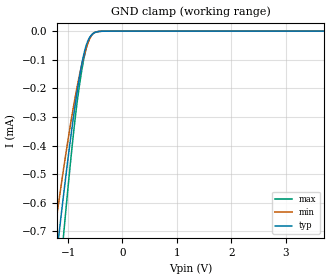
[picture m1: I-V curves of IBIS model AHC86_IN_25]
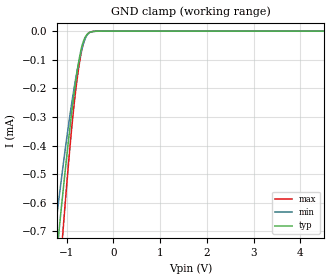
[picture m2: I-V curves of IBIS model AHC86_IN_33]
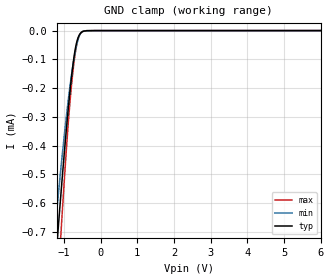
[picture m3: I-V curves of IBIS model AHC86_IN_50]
| TEXAS INSTRUMENTS INCORPORATED
| Standard Linear and Logic Group
| IBIS Model of SN74AHC86
| QUADRUPLE 2-INPUT EXCLUSIVE-OR GATES
| This file contains package information for the following:
|  SOIC 14-pin (D) package as [Component] AHC86_PKG_D
|  SSOP 14-pin (DB) package as [Component] AHC86_PKG_DB
|  TVSOP 14-pin (DGV) package as [Component] AHC86_PKG_DGV
|  PDIP 14-pin (N) package as [Component] AHC86_PKG_N
|  TSSOP 14-pin (PW) package as [Component] AHC86_PKG_PW
| This device can be powered at the following Vccs:
|  2.5 volt Vcc
|  3.3 volt Vcc
|  5.0 volt Vcc
| This file provides unique models under the [Model Selector] for each Vcc.
| For operation at a specific Vcc, select the appropriate model after each
| [Model Selector] keyword.
[IBIS Ver]   3.2
[Comment char]  |_char
[File Name]   ahc86.ibs
[File Rev]   1.1 | B_die
[Date]   October 12, 2000
[Source]   Data created from TI-SPICE simulations at TI-SLL.
[Notes]   The following is an IBIS list for the AHC86_PKG.
   Please contact sllibis@ti.com with questions and
   comments concerning SLL IBIS models.
   -To comply with the data sheet we omitted the Vref
   and Rref from the Output Model
   -As there is no power clamp diode in the Input Model,
   we removed the Pwr Clamp table data from the Input Models
[Disclaimer] Property of Texas Instruments Incorporated.  Unauthorized
   reproduction and/or distribution is strictly prohibited.
   This product is protected under copyright law.
   Created  2000, (C) Copyright  2000, Texas Instruments Inc.,
   All Rights Reserved
   UNLESS THERE IS A SIGNED, WRITTEN AGREEMENT TO THE
   CONTRARY, TEXAS INSTRUMENTS (TI) IS PROVIDING THE IBIS
   MODELS  AND WITHOUT ANY WARRANTY, EXPRESSED OR
   IMPLIED.  TI assumes no liability for:
   1) the accuracy of the IBIS models provided to your
   company;
   2) the proper functioning of these IBIS Models in your
   design or for any resulting applications; or
   3) infringement of patents, copyrights or intellectual
   property rights resulting from your use of these IBIS
   models.
   TI provides IBIS Models as a service to our customers.
   You and your company shall not distribute, sell or give
   these models to anyone else without prior written
   permission from TI.
   TI reserves the right to make changes to our products or
   to discontinue any semiconductor product or service
   without notice, and advises our customers to obtain the
   latest version of relevant information to verify, before
   placing orders, that the information being relied on is
   current.
   Please be aware that your receipt and use of the IBIS
   information provided shall serve as acceptance of these
   terms and conditions.  If you do not accept these terms,
   you should return or destroy the IBIS models and any
   other accompanying information immediately.
| Component AHC86_PKG_D 14-pin SOIC
[Component]   AHC86_PKG_D
[Manufacturer]   Texas Instruments, Inc.
[Package]
|   typ   min   max
R_pkg   3.100e-02   2.800e-02   3.400e-02
L_pkg   3.109e-09   2.462e-09   3.889e-09
C_pkg   4.730e-13   3.630e-13   6.280e-13
[Pin]   signal_name   model_name   R_pin   L_pin   C_pin
1   1A   AHC86_IN   3.300e-02   3.854e-09   6.220e-13
2   1B   AHC86_IN   3.200e-02   3.188e-09   4.730e-13
3   1Y   AHC86_OUT   2.800e-02   2.462e-09   3.770e-13
4   2A   AHC86_IN   3.100e-02   2.596e-09   3.630e-13
5   2B   AHC86_IN   2.800e-02   2.521e-09   3.720e-13
6   2Y   AHC86_OUT   3.400e-02   3.250e-09   4.760e-13
7   GND   GND   3.400e-02   3.889e-09   6.280e-13
8   3Y   AHC86_OUT   3.400e-02   3.889e-09   6.280e-13
9   3A   AHC86_IN   3.400e-02   3.250e-09   4.760e-13
10   3B   AHC86_IN   2.800e-02   2.521e-09   3.720e-13
11   4Y   AHC86_OUT   3.100e-02   2.596e-09   3.640e-13
12   4A   AHC86_IN   2.800e-02   2.462e-09   3.770e-13
13   4B   AHC86_IN   3.200e-02   3.188e-09   4.730e-13
14   VCC   POWER   3.300e-02   3.854e-09   6.220e-13
| Component AHC86_PKG_DB 14-pin SSOP
[Component]   AHC86_PKG_DB
[Manufacturer]   Texas Instruments, Inc.
[Package]
|   typ   min   max
R_pkg   4.400e-02   4.100e-02   4.600e-02
L_pkg   3.551e-09   3.258e-09   3.927e-09
C_pkg   4.020e-13   3.600e-13   4.210e-13
[Pin]   signal_name   model_name   R_pin   L_pin   C_pin
1   1A   AHC86_IN   4.600e-02   3.927e-09   4.080e-13
2   1B   AHC86_IN   4.400e-02   3.587e-09   4.210e-13
3   1Y   AHC86_OUT   4.100e-02   3.289e-09   3.980e-13
4   2A   AHC86_IN   4.200e-02   3.258e-09   3.600e-13
5   2B   AHC86_IN   4.100e-02   3.286e-09   4.030e-13
6   2Y   AHC86_OUT   4.400e-02   3.586e-09   4.210e-13
7   GND   GND   4.600e-02   3.927e-09   4.080e-13
8   3Y   AHC86_OUT   4.600e-02   3.927e-09   4.080e-13
9   3A   AHC86_IN   4.400e-02   3.586e-09   4.210e-13
10   3B   AHC86_IN   4.100e-02   3.286e-09   4.030e-13
11   4Y   AHC86_OUT   4.300e-02   3.258e-09   3.600e-13
12   4A   AHC86_IN   4.100e-02   3.289e-09   3.980e-13
13   4B   AHC86_IN   4.400e-02   3.587e-09   4.210e-13
14   VCC   POWER   4.600e-02   3.927e-09   4.080e-13
| Component AHC86_PKG_DGV 14-pin TVSOP
[Component]   AHC86_PKG_DGV
[Manufacturer]   Texas Instruments, Inc.
[Package]
|   typ   min   max
R_pkg   3.500e-02   2.000e-02   4.500e-02
L_pkg   2.499e-09   2.077e-09   2.966e-09
C_pkg   3.610e-13   3.050e-13   4.160e-13
[Pin]   signal_name   model_name   R_pin   L_pin   C_pin
1   1A   AHC86_IN   2.700e-02   2.717e-09   3.730e-13
2   1B   AHC86_IN   3.700e-02   2.434e-09   3.980e-13
3   1Y   AHC86_OUT   3.400e-02   2.200e-09   3.160e-13
4   2A   AHC86_IN   2.000e-02   2.077e-09   3.090e-13
5   2B   AHC86_IN   3.000e-02   2.147e-09   3.050e-13
6   2Y   AHC86_OUT   4.200e-02   2.580e-09   4.080e-13
7   GND   GND   3.900e-02   2.921e-09   3.850e-13
8   3Y   AHC86_OUT   3.300e-02   2.841e-09   3.800e-13
9   3A   AHC86_IN   4.200e-02   2.611e-09   4.100e-13
10   3B   AHC86_IN   3.800e-02   2.331e-09   3.290e-13
11   4Y   AHC86_OUT   2.600e-02   2.223e-09   3.190e-13
12   4A   AHC86_IN   3.400e-02   2.259e-09   3.130e-13
13   4B   AHC86_IN   4.500e-02   2.681e-09   4.160e-13
14   VCC   POWER   4.200e-02   2.966e-09   3.860e-13
| Component AHC86_PKG_N 14-pin PDIP
[Component]   AHC86_PKG_N
[Manufacturer]   Texas Instruments, Inc.
[Package]
|   typ   min   max
R_pkg   4.500e-02   3.700e-02   6.300e-02
L_pkg   5.407e-09   3.922e-09   6.942e-09
C_pkg   3.890e-13   2.050e-13   6.040e-13
[Pin]   signal_name   model_name   R_pin   L_pin   C_pin
1   1A   AHC86_IN   6.300e-02   6.942e-09   6.040e-13
2   1B   AHC86_IN   3.700e-02   6.200e-09   4.060e-13
3   1Y   AHC86_OUT   4.200e-02   4.389e-09   3.220e-13
4   2A   AHC86_IN   3.800e-02   3.922e-09   2.050e-13
5   2B   AHC86_IN   3.900e-02   4.301e-09   2.980e-13
6   2Y   AHC86_OUT   3.800e-02   5.329e-09   3.560e-13
7   GND   GND   5.300e-02   6.510e-09   5.440e-13
8   3Y   AHC86_OUT   5.300e-02   6.437e-09   5.390e-13
9   3A   AHC86_IN   3.900e-02   5.352e-09   3.470e-13
10   3B   AHC86_IN   4.200e-02   4.473e-09   2.970e-13
11   4Y   AHC86_OUT   4.400e-02   4.326e-09   2.250e-13
12   4A   AHC86_IN   4.200e-02   4.295e-09   2.800e-13
13   4B   AHC86_IN   4.200e-02   6.318e-09   4.180e-13
14   VCC   POWER   6.100e-02   6.900e-09   6.030e-13
| Component AHC86_PKG_PW 14-pin TSSOP
[Component]   AHC86_PKG_PW
[Manufacturer]   Texas Instruments, Inc.
[Package]
|   typ   min   max
R_pkg   3.200e-02   2.900e-02   3.500e-02
L_pkg   2.378e-09   2.170e-09   2.680e-09
C_pkg   3.140e-13   2.700e-13   3.350e-13
[Pin]   signal_name   model_name   R_pin   L_pin   C_pin
1   1A   AHC86_IN   3.300e-02   2.618e-09   3.300e-13
2   1B   AHC86_IN   3.100e-02   2.313e-09   3.170e-13
3   1Y   AHC86_OUT   3.000e-02   2.310e-09   3.140e-13
4   2A   AHC86_IN   3.100e-02   2.173e-09   2.720e-13
5   2B   AHC86_IN   3.000e-02   2.204e-09   3.090e-13
6   2Y   AHC86_OUT   3.200e-02   2.315e-09   3.170e-13
7   GND   GND   3.500e-02   2.680e-09   3.350e-13
8   3Y   AHC86_OUT   3.300e-02   2.640e-09   3.330e-13
9   3A   AHC86_IN   3.400e-02   2.347e-09   3.190e-13
10   3B   AHC86_IN   2.900e-02   2.277e-09   3.130e-13
11   4Y   AHC86_OUT   3.100e-02   2.170e-09   2.700e-13
12   4A   AHC86_IN   3.100e-02   2.244e-09   3.110e-13
13   4B   AHC86_IN   3.300e-02   2.343e-09   3.210e-13
14   VCC   POWER   3.500e-02   2.657e-09   3.320e-13
| Model AHC86_IN
[Model Selector]   AHC86_IN
AHC86_IN_25   2.5 volt Vcc
AHC86_IN_33   3.3 volt Vcc
AHC86_IN_50   5.0 volt Vcc
| Model AHC86_OUT
[Model Selector]   AHC86_OUT
AHC86_OUT_25   2.5 volt Vcc
AHC86_OUT_33   3.3 volt Vcc
AHC86_OUT_50   5.0 volt Vcc
| Models and submodels in the file (6): AHC86_IN_25 (Input), AHC86_IN_33 (Input), AHC86_IN_50 (Input), AHC86_OUT_25 (Output), AHC86_OUT_33 (Output), AHC86_OUT_50 (Output)
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[Model]   AHC86_IN_25
Model_type  Input
Vinl =   0.7
Vinh =   1.7
| variable   typ   min   max
C_comp   0.82pF   0.77pF   0.88pF
[Temperature Range]   40   100   -40
| Ambient temperature   25   85   -40
[Voltage range]   2.5   2.3   2.7
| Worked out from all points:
|   GND clamp passes 1 mA (typ) near -1.34 V on its own axis
[GND Clamp]
| AHC86_IN_25
|   Voltage   I(typ)   I(min)   I(max)
-2.51V    -3.318mA   -2.676mA   -4.056mA
-1.27V    -883uA     -731.2uA   -1.114mA
-1.215V   -789.1uA   -655.8uA   -993.6uA
-1.16V    -697.2uA   -581.9uA   -874.9uA
-1.105V   -607.5uA   -509.8uA   -758.5uA
-1.065V   -543.9uA   -458.6uA   -675.4uA
-880mV    -271.8uA   -241.5uA   -322.3uA
-805mV    -177.1uA   -166.7uA   -208.1uA
-740mV    -107.3uA   -110.6uA   -127.9uA
-620mV    -27.63uA   -34.06uA   -32.65uA
-485mV    -3.243uA   -2.794uA   -2.75uA
7.555V    17.81nA    515.6pA    227.5nA
[Model]   AHC86_IN_33
Model_type  Input
Vinl =   0.9
Vinh =   2.1
| variable   typ   min   max
C_comp   0.82pF   0.77pF   0.89pF
[Temperature Range]   40   100   -40
| Ambient temperature   25   85   -40
[Voltage range]   3.3   3   3.6
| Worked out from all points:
|   GND clamp passes 1 mA (typ) near -1.34 V on its own axis
[GND Clamp]
| AHC86_IN_33
|   Voltage   I(typ)   I(min)   I(max)
-3.4V     -5.269mA   -4.235mA   -6.279mA
-1.27V    -883uA     -731.2uA   -1.114mA
-1.215V   -789.1uA   -655.8uA   -993.6uA
-1.16V    -697.2uA   -581.9uA   -875uA
-1.105V   -607.6uA   -509.8uA   -758.5uA
-1.065V   -543.9uA   -458.6uA   -675.4uA
-880mV    -271.8uA   -241.5uA   -322.3uA
-805mV    -177.1uA   -166.7uA   -208.1uA
-740mV    -107.3uA   -110.6uA   -127.9uA
-620mV    -27.63uA   -34.06uA   -32.66uA
-485mV    -3.244uA   -2.794uA   -2.754uA
7.975V    21.54nA    562.3pA    257.8nA
[Model]   AHC86_IN_50
Model_type  Input
Vinl =   1.35
Vinh =   3.85
| variable   typ   min   max
C_comp   0.83pF   0.76pF   0.95pF
[Temperature Range]   40   100   -40
| Ambient temperature   25   85   -40
[Voltage range]   5   4.5   5.5
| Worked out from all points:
|   GND clamp passes 1 mA (typ) near -1.34 V on its own axis
[GND Clamp]
| AHC86_IN_50
|   Voltage   I(typ)   I(min)   I(max)
-5V       -8.966mA   -7.191mA   -10.36mA
-1.27V    -883uA     -731.2uA   -1.114mA
-1.215V   -789.1uA   -655.8uA   -993.6uA
-1.16V    -697.2uA   -581.9uA   -875uA
-1.105V   -607.6uA   -509.8uA   -758.5uA
-1.065V   -543.9uA   -458.6uA   -675.4uA
-880mV    -271.8uA   -241.5uA   -322.3uA
-805mV    -177.1uA   -166.7uA   -208.2uA
-740mV    -107.3uA   -110.6uA   -127.9uA
-620mV    -27.63uA   -34.06uA   -32.68uA
-485mV    -3.248uA   -2.795uA   -2.776uA
6.005V    7.954nA    367.8pA    85.01nA
